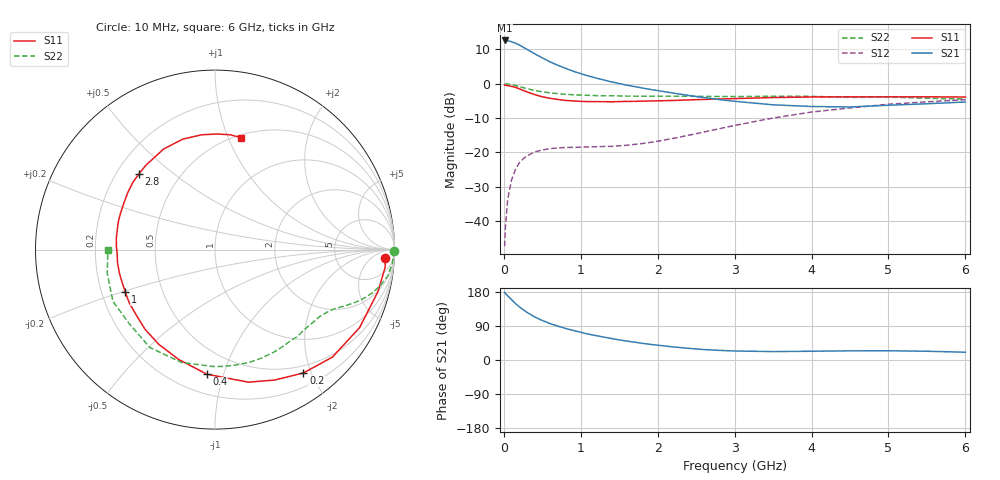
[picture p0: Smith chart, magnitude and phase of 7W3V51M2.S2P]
! Infineon Technologies  Discrete & RF Semiconductors
! BFS17W
! Si NPN RF Bipolar Junction Transistor in SOT323
! VCE = 3.5 V  IC = 1.2 mA
! Common Emitter S-Parameters:  August  1999
# GHz  S  MA  R  50
!  f  S11  S21  S12  S22
! GHz  MAG  ANG  MAG  ANG  MAG  ANG  MAG  ANG
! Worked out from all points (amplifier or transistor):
!   36 points, 10 MHz to 6 GHz, reference 50 ohm
!   highest |S21| = 12.6 dB at 10 MHz (marker M1)
!   |S21| within 3 dB of that: start of sweep to 332.8 MHz
!   unconditionally stable (mu >= 1): 980.3 MHz to end of sweep
!   at 250 MHz: K = 0.28, MSG = 16.3 dB, |S12| = -21.9 dB
!   at 1.4 GHz: K = 1.29, MAG = 6.1 dB, |S12| = -18.2 dB
!   at 6 GHz: K = 1.10, MAG = -2.3 dB, |S12| = -4.7 dB
!   S11 on the Smith chart (normalised r, x): 10 MHz: 20, -19; 200 MHz: 0.39, -1.88; 400 MHz: 0.33, -0.88; 1 GHz: 0.30, -0.21; 2.8 GHz: 0.29, +0.38; 6 GHz: 0.52, +1.11
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0.01  0.9498 -2.8  4.272 178.6  0.0043 82.8  1 -0.4
0.02  0.9529 -6.0  4.26 175.9  0.008 89.1  0.9939 -1.8
0.05  0.9378 -14.5  4.237 169.3  0.0206 81.6  0.9909 -4.4
0.1  0.9153 -28.4  4.091 159.3  0.0395 75.1  0.9745 -8.6
0.15  0.887 -42.5  3.914 149.3  0.0561 66.2  0.943 -12.2
0.2  0.8454 -54.4  3.676 140.6  0.0703 60.6  0.9117 -15.2
0.25  0.7993 -65.4  3.417 132.8  0.0803 54.8  0.8786 -17.7
0.3  0.7615 -75.9  3.176 125.8  0.0891 50.4  0.8497 -19.7
0.4  0.6958 -93.7  2.736 113.7  0.1015 43.3  0.7995 -22.8
0.5  0.6446 -108.3  2.378 104.3  0.1084 38.9  0.7632 -25.0
0.6  0.6137 -120.7  2.084 96.2  0.1132 36.1  0.7366 -26.9
0.7  0.5908 -131.3  1.861 89.5  0.1161 34.4  0.7173 -28.9
0.8  0.5707 -140.1  1.681 83.4  0.1178 33.4  0.7023 -31.0
1  0.5535 -154.5  1.401 73.2  0.1191 33.9  0.6849 -35.0
1.1  0.5486 -161.6  1.299 68.3  0.1202 34.5  0.6774 -37.5
1.6  0.5532 173.7  0.953 49.9  0.1269 43.7  0.6601 -50.1
2.2  0.5706 152.7  0.732 34.5  0.1598 57.3  0.6578 -67.0
2.8  0.5985 134.9  0.588 25.4  0.2209 63.3  0.6526 -85.2
3.5  0.6294 117.0  0.493 22.2  0.317 61.3  0.6558 -106.6
4.5  0.644 96.5  0.459 24.2  0.4439 49.3  0.6317 -139.2
5.5  0.6454 82.4  0.511 23.1  0.5461 36.2  0.6149 -167.5
6  0.6403 77.1  0.542 20.5  0.5848 30.1  0.5968 -179.9
